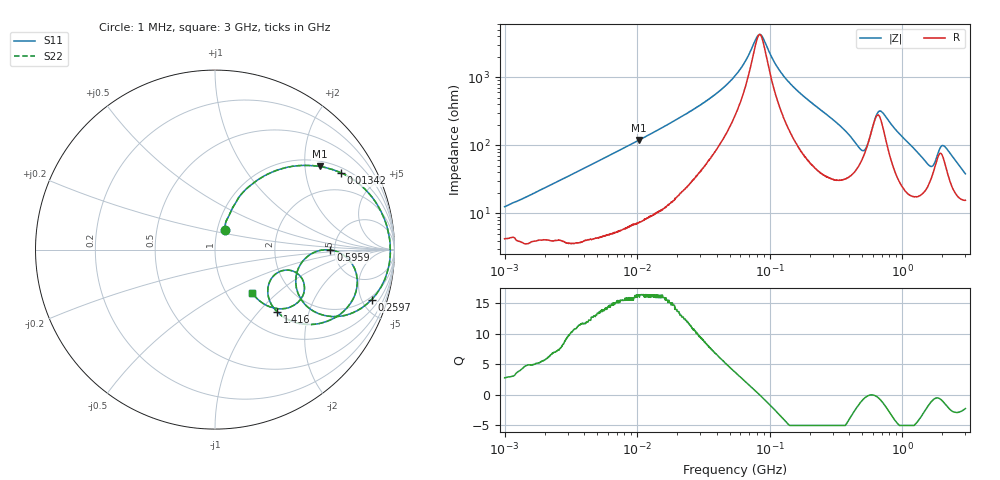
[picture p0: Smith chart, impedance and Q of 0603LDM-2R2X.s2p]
!s-Parameter Generated by FASTRON Sdn. Bhd.
!FASTRON P/N : 0603LDM-2R2X
!Keysight Technologies: E4991B_MY54100416_A.01.15
!Date: Thu Nov 27 16:25:06 2025
!Version  :Rev00  Thu Nov 27 16:25:06 2025
!Data & Calibration Information:
!Freq  S11  S21  S12  S22
!PortZ  Port1:50+j0  Port2:50+j0
!When reading reference impedance value at option line is always used.
! Remarks : This data is being provided solely for informational purposes.
# Hz S dB R 50
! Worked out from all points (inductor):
!   1601 points, 1 MHz to 3 GHz, reference 50 ohm
!   read as one part in series: L = 1.87 uH near 1.128 MHz
!   highest Q = 16.4 at 10.35 MHz (marker M1), where L = 1.84 uH
!   self-resonance near 84.06 MHz
!   S11 on the Smith chart (normalised r, x): 1 MHz: 1.09, +0.24; 13.42 MHz: 1.19, +3.14; 259.7 MHz: 1.71, -5.94; 595.9 MHz: 4.60, -0.04; 1.416 GHz: 1.38, -1.27; 3 GHz: 1.31, -0.70
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1000000  -18.40 63.8  -0.41 -6.5  -0.41 -6.5  -18.40 63.8
3804036  -8.14 62.1  -1.04 -23.0  -1.04 -23.0  -8.14 62.1
1.034868e7  -2.55 38.4  -4.12 -48.1  -4.12 -48.1  -2.55 38.4
1.342429e7  -1.71 31.4  -5.64 -55.0  -5.64 -55.0  -1.71 31.4
1.447069e7  -1.52 29.5  -6.13 -56.9  -6.13 -56.9  -1.52 29.5
3.254976e7  -0.43 12.5  -13.20 -70.9  -13.20 -70.9  -0.43 12.5
5.504702e7  -0.25 5.1  -20.80 -69.7  -20.80 -69.7  -0.25 5.1
8.507507e7  -0.20 -0.1  -32.80 6.0  -32.80 6.0  -0.20 -0.1
1.263238e8  -0.23 -5.0  -20.80 70.6  -20.80 70.6  -0.23 -5.0
2.083556e8  -0.47 -13.0  -12.90 70.0  -12.90 70.0  -0.47 -13.0
2.596726e8  -0.76 -17.7  -10.30 65.4  -10.30 65.4  -0.76 -17.7
4.177151e8  -3.16 -31.4  -5.27 41.7  -5.27 41.7  -3.16 -31.4
5.077325e8  -6.39 -19.9  -4.84 16.5  -4.84 16.5  -6.39 -19.9
5.959055e8  -3.84 -0.2  -8.94 0.4  -8.94 0.4  -3.84 -0.2
6.753166e8  -2.09 -7.9  -12.20 25.9  -12.20 25.9  -2.09 -7.9
7.925923e8  -1.75 -19.6  -8.93 49.9  -8.93 49.9  -1.75 -19.6
1.070143e9  -3.06 -36.1  -4.47 43.8  -4.47 43.8  -3.06 -36.1
1.416254e9  -6.17 -45.1  -2.62 28.1  -2.62 28.1  -6.17 -45.1
1.695807e9  -9.05 -28.1  -2.99 13.6  -2.99 13.6  -9.05 -28.1
2.050964e9  -5.22 -25.1  -5.12 24.8  -5.12 24.8  -5.22 -25.1
2.371269e9  -6.05 -41.5  -3.00 27.8  -3.00 27.8  -6.05 -41.5
3e9  -10.00 -49.1  -1.64 16.8  -1.64 16.8  -10.00 -49.1
